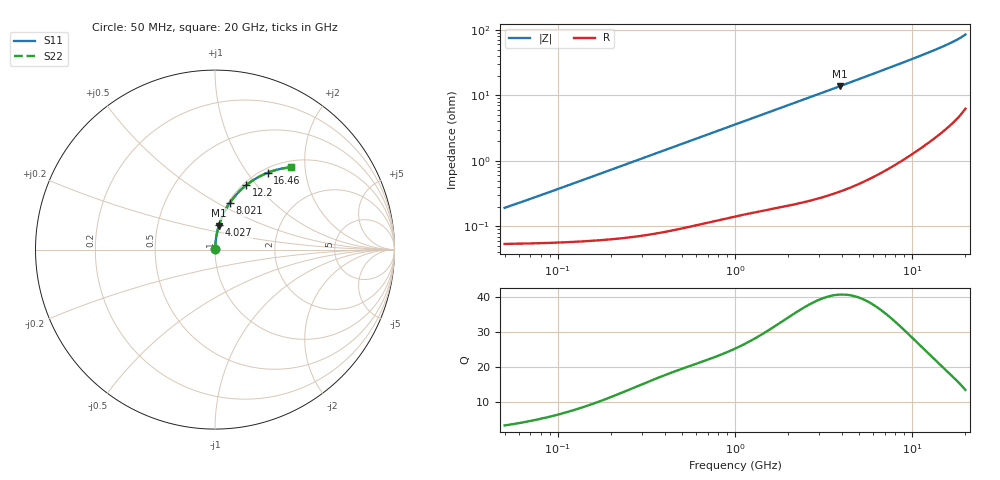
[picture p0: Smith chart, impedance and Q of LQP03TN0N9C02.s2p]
!Murata Part Number: LQP03TN0N9C02
!These Parameters are Measured in Series Mode Connection
!  o--[Z]--o
!Port1  Port2
!  o-------o
!Freq. Start=50[MHz] Stop=20[GHz], 401[Steps]
# Hz S RI R 50
!Freq.(Hz) S11(Real) S11(Imag) S21(Real) S21(Imag) S12(Real) S12(Imag) S22(Real) S22(Imag)
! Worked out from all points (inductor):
!   401 points, 50 MHz to 20 GHz, reference 50 ohm
!   read as one part in series: L = 586 pH near 51.52 MHz
!   highest Q = 40.5 at 3.908 GHz (marker M1), where L = 560 pH
!   S11 on the Smith chart (normalised r, x): 50 MHz: 1.00, +0.00; 4.027 GHz: 1.01, +0.28; 8.021 GHz: 1.02, +0.57; 12.2 GHz: 1.04, +0.88; 16.46 GHz: 1.07, +1.25; 20 GHz: 1.13, +1.69
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5e7  0.000543 0.00184  0.9995 -0.00184  0.9995 -0.00184  0.000543 0.00184
5.152053e7  0.000544 0.0019  0.9995 -0.0019  0.9995 -0.0019  0.000544 0.0019
6.746414e7  0.000554 0.00248  0.9994 -0.00248  0.9994 -0.00248  0.000554 0.00248
1.364002e8  0.000614 0.00499  0.9994 -0.00499  0.9994 -0.00499  0.000614 0.00499
3.721004e8  0.000974 0.0135  0.999 -0.0135  0.999 -0.0135  0.000974 0.0135
6.380365e8  0.0016 0.0229  0.9984 -0.0229  0.9984 -0.0229  0.0016 0.0229
1e9  0.00268 0.0355  0.9973 -0.0355  0.9973 -0.0355  0.00268 0.0355
1.714689e9  0.00554 0.0601  0.9945 -0.0601  0.9945 -0.0601  0.00554 0.0601
2.728004e9  0.0116 0.0947  0.9884 -0.0947  0.9884 -0.0947  0.0116 0.0947
3.908127e9  0.0217 0.1341  0.9783 -0.1341  0.9783 -0.1341  0.0217 0.1341
4.026975e9  0.023 0.138  0.977 -0.138  0.977 -0.138  0.023 0.138
5.598765e9  0.042 0.1881  0.958 -0.1881  0.958 -0.1881  0.042 0.1881
7.442007e9  0.0712 0.2429  0.9288 -0.2429  0.9288 -0.2429  0.0712 0.2429
8.020766e9  0.0817 0.2591  0.9183 -0.2591  0.9183 -0.2591  0.0817 0.2591
1.004137e10  0.123 0.3112  0.877 -0.3112  0.877 -0.3112  0.123 0.3112
1.115139e10  0.1483 0.3367  0.8517 -0.3367  0.8517 -0.3367  0.1483 0.3367
1.220001e10  0.1738 0.3588  0.8262 -0.3588  0.8262 -0.3588  0.1738 0.3588
1.438523e10  0.2316 0.3984  0.7684 -0.3984  0.7684 -0.3984  0.2316 0.3984
1.646126e10  0.2928 0.428  0.7072 -0.428  0.7072 -0.428  0.2928 0.428
1.800918e10  0.3441 0.4448  0.6559 -0.4448  0.6559 -0.4448  0.3441 0.4448
1.940974e10  0.3977 0.4556  0.6023 -0.4556  0.6023 -0.4556  0.3977 0.4556
2e10  0.4238 0.4585  0.5762 -0.4585  0.5762 -0.4585  0.4238 0.4585
